FUNCTION FC 36 : VOID
TITLE =LOAD PARAMETERS FOR MACHINE LINE
VERSION : 0.1

BEGIN
NETWORK
TITLE =LOAD PARAMETERS FROM RECIPE

      U     M    121.1;
      U     A     47.6;
      UN    M     33.3;
      UN    M     33.4;
      SPB   M001;
      SPA   M002;

M001: L     DB16.DBD   90;
      T     DB14.DBD  282;
      L     DB16.DBD   98;
      T     DB14.DBD  142;
      L     DB16.DBD  134;
      T     DB14.DBD  134;
      L     DB16.DBD  138;
      T     DB14.DBD  138;
      S     M    100.0;
M002: NOP   0;
NETWORK
TITLE =LOAD PARAMETERS FROM RECIPE

      U     M     47.0;
      U     A     47.6;
      UN    M     33.3;
      UN    M     33.4;
      FP    M     47.1;
      SPB   M003;
      SPA   M004;

M003: L     DB14.DBD  274;
      T     DB14.DBD  282;
      L     DB14.DBD  278;
      T     DB14.DBD  142;
      L     DB14.DBD  266;
      T     DB14.DBD  134;
      L     DB14.DBD  270;
      T     DB14.DBD  138;
      S     M    100.0;
M004: NOP   0;


NETWORK
TITLE =LOAD PARAMETERS AFTER START
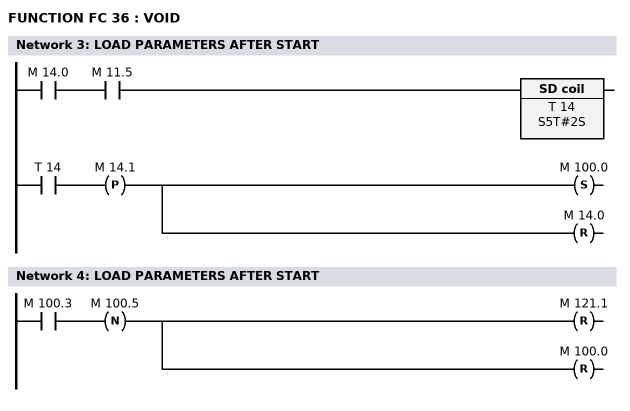
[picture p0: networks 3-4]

      U     M     14.0;
      U     M     11.5;
      L     S5T#2S;
      SE    T     14;

      U     T     14;
      FP    M     14.1;
      S     M    100.0;
      R     M     14.0;

NETWORK
TITLE =LOAD PARAMETERS AFTER START

      U     M    100.3;
      FN    M    100.5;
      R     M    121.1;
      R     M    100.0;
END_FUNCTION

